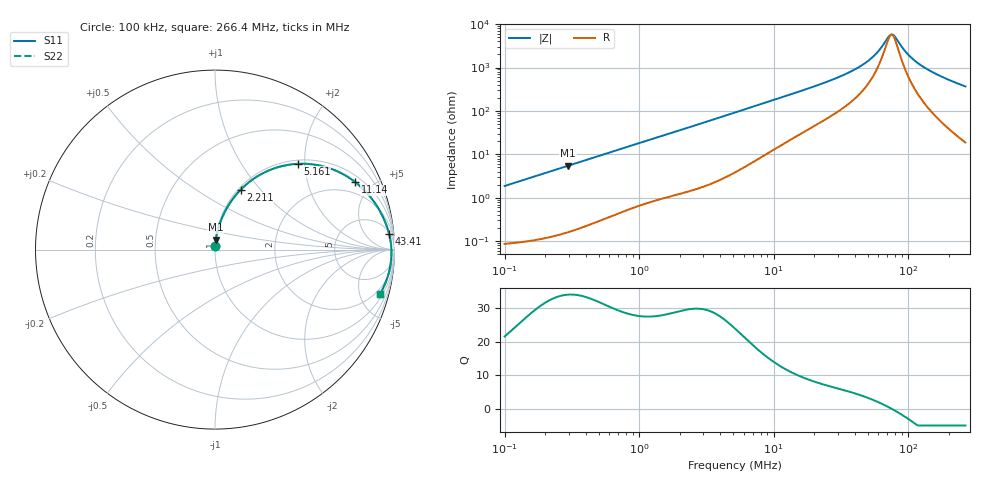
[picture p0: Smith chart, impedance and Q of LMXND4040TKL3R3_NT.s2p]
! LMXND4040TKL3R3_NT  S-PARAMETER MODEL  ( Standard Model )
! Model Generated by TAIYO YUDEN Corporation (https://www.yuden.co.jp/en/)
! Version 1.0
! TAIYO YUDEN Control No. 20251120
! Copyright(c) 2025 TAIYO YUDEN CO.,LTD. All Rights Reserved.
! Product Description (link to TY-COMPAS)
! https://ds.yuden.co.jp/TYCOMPAS/or/detail?pn=LMXND4040TKL3R3MNT&u=M
! Products Name : Inductors
! Characteristics :
!  Inductance : 3.3 [uH] , SRF(min) : 45 [MHz] , DC Resistance(max) : 0.066 [Ohm]
!  Rated Current : Saturation  2300 [mA] , Temp Rise  2500 [mA] (40 [degC])
!  Case Size : 4.0 x 4.0 / 0.157 x 0.157 [mm/inch] , Thickness : 1.8 / 0.071 [mm/inch]
!  (Conditions: Temperature = 25 [degC] , DC Bias Current = 0 [A])
! External Node Assignments :
!  1  o---GGG---o  2
! GND o---------o GND
! Frequency Range : 0.1MHz  -  266.375554MHz  [ 402 STEP ]
# MHz S RI R 50
! Freq[MHz].  S11 Real  S11 Imag  S21 Real  S21 Imag  S12 Real  S12 Imag  S22 Real  S22 Imag
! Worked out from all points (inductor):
!   401 points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, 100 kHz to 266.4 MHz, reference 50 ohm
!   read as one part in series: L = 2.96 uH near 104 kHz
!   highest Q = 34.1 at 295.8 kHz (marker M1), where L = 2.95 uH
!   self-resonance near 73.94 MHz
!   S11 on the Smith chart (normalised r, x): 100 kHz: 1.00, +0.04; 2.211 MHz: 1.03, +0.79; 5.161 MHz: 1.08, +1.84; 11.14 MHz: 1.31, +3.98; 43.41 MHz: 6, +20; 266.4 MHz: 1.37, -7.30
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0.1  0.00121 0.0186  0.9988 -0.0186  0.9988 -0.0186  0.00121 0.0186
0.295805  0.00459 0.0545  0.9954 -0.0545  0.9954 -0.0545  0.00459 0.0545
0.374775  0.0068 0.0687  0.9932 -0.0687  0.9932 -0.0687  0.0068 0.0687
0.762193  0.0236 0.1353  0.9764 -0.1353  0.9764 -0.1353  0.0236 0.1353
1.404561  0.0674 0.2334  0.9326 -0.2334  0.9326 -0.2334  0.0674 0.2334
2.210582  0.1428 0.3334  0.8572 -0.3334  0.8572 -0.3334  0.1428 0.3334
3.279301  0.2611 0.4225  0.7389 -0.4225  0.7389 -0.4225  0.2611 0.4225
5.161158  0.4599 0.478  0.5401 -0.478  0.5401 -0.478  0.4599 0.478
5.26394  0.4693 0.4784  0.5307 -0.4784  0.5307 -0.4784  0.4693 0.4784
7.360282  0.6266 0.457  0.3734 -0.457  0.3734 -0.457  0.6266 0.457
11.13609  0.7817 0.3759  0.2183 -0.3759  0.2183 -0.3759  0.7817 0.3759
19.34272  0.9009 0.2447  0.0991 -0.2447  0.0991 -0.2447  0.9009 0.2447
31.04897  0.9505 0.1479  0.0495 -0.1479  0.0495 -0.1479  0.9505 0.1479
43.41409  0.9698 0.0889  0.0302 -0.0889  0.0302 -0.0889  0.9698 0.0889
57.21672  0.9789 0.0437  0.0211 -0.0437  0.0211 -0.0437  0.9789 0.0437
72.49162  0.9827 0.006  0.0173 -0.006  0.0173 -0.006  0.9827 0.006
75.40763  0.9829 -0.000293  0.0171 0.000293  0.0171 0.000293  0.9829 -0.000293
78.44093  0.9831 -0.00661  0.0169 0.00661  0.0169 0.00661  0.9831 -0.00661
99.38196  0.9823 -0.0453  0.0177 0.0453  0.0177 0.0453  0.9823 -0.0453
128.421  0.9769 -0.09  0.0231 0.09  0.0231 0.09  0.9769 -0.09
179.5642  0.9605 -0.1559  0.0395 0.1559  0.0395 0.1559  0.9605 -0.1559
266.3756  0.9195 -0.2476  0.0805 0.2476  0.0805 0.2476  0.9195 -0.2476
